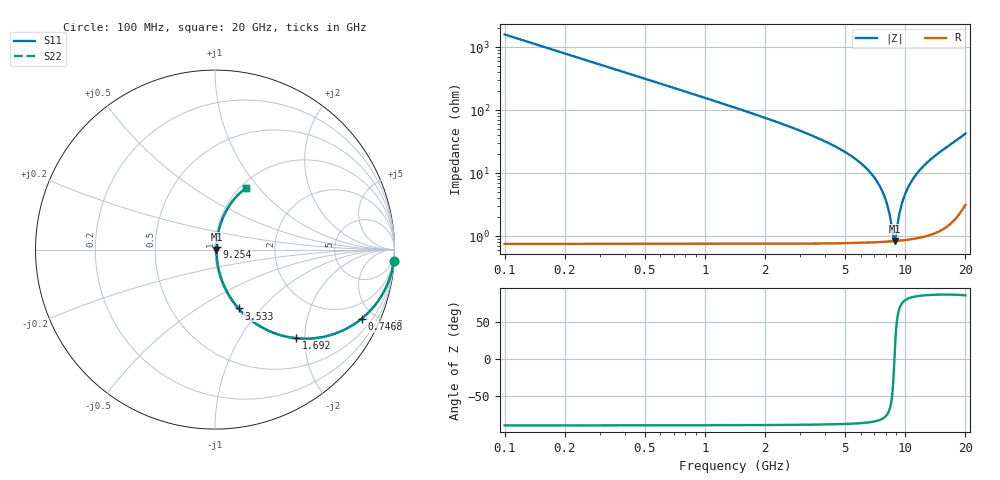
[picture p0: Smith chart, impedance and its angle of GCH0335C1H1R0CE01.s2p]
!Murata Part Number: GCH0335C1H1R0CE01
!These Parameters are Measured in Series Mode Connection
!Data Generated on Mar 13, 2026
!  o--ll--o
!Port1  Port2
!  o------o
!Operation Temp=25[degC], DC Bias Voltage=0[V]
!Freq. Start=100[MHz] Stop=20[GHz] 401[Steps]
# Hz S RI R 50
!Freq.(Hz) S11(Real) S11(Imag) S21(Real) S21(Imag) S12(Real) S12(Imag) S22(Real) S22(Imag)
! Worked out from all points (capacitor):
!   401 points, 100 MHz to 20 GHz, reference 50 ohm
!   read as one part in series: C = 1 pF near 199.5 MHz
!   lowest |Z| = 840 mohm at 8.856 GHz (marker M1)
!   series resonance near 8.845 GHz, so ESL is about 320 pH
!   S11 on the Smith chart (normalised r, x): 100 MHz: 1, -32; 746.8 MHz: 1.02, -4.23; 1.692 GHz: 1.02, -1.81; 3.533 GHz: 1.02, -0.76; 9.254 GHz: 1.02, +0.03; 20 GHz: 1.06, +0.85
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1e8  0.996 -0.0626  0.00396 0.0626  0.00396 0.0626  0.996 -0.0626
2.99e8  0.9656 -0.1816  0.0344 0.1816  0.0344 0.1816  0.9656 -0.1816
3.985e8  0.9404 -0.2358  0.0596 0.2358  0.0596 0.2358  0.9404 -0.2358
7.4675e8  0.8166 -0.3852  0.1834 0.3852  0.1834 0.3852  0.8166 -0.3852
1.1945e9  0.6306 -0.4797  0.3694 0.4797  0.3694 0.4797  0.6306 -0.4797
1.692e9  0.4518 -0.4935  0.5482 0.4935  0.5482 0.4935  0.4518 -0.4935
2.488e9  0.2611 -0.4328  0.7389 0.4328  0.7389 0.4328  0.2611 -0.4328
3.43325e9  0.1399 -0.3373  0.8601 0.3373  0.8601 0.3373  0.1399 -0.3373
3.53275e9  0.1312 -0.3277  0.8688 0.3277  0.8688 0.3277  0.1312 -0.3277
6.7665e9  0.0174 -0.0965  0.9826 0.0965  0.9826 0.0965  0.0174 -0.0965
7.9605e9  0.00959 -0.0381  0.9904 0.0381  0.9904 0.0381  0.00959 -0.0381
8.3585e9  0.00863 -0.0205  0.9914 0.0205  0.9914 0.0205  0.00863 -0.0205
8.7565e9  0.00831 -0.00366  0.9917 0.00366  0.9917 0.00366  0.00831 -0.00366
8.856e9  0.00832 0.000444  0.9917 -0.000444  0.9917 -0.000444  0.00832 0.000444
8.9555e9  0.00837 0.00451  0.9916 -0.00451  0.9916 -0.00451  0.00837 0.00451
9.254e9  0.0087 0.0165  0.9913 -0.0165  0.9913 -0.0165  0.0087 0.0165
9.60225e9  0.00943 0.03  0.9906 -0.03  0.9906 -0.03  0.00943 0.03
1.005e10  0.0109 0.0468  0.9891 -0.0468  0.9891 -0.0468  0.0109 0.0468
1.13435e10  0.0178 0.0923  0.9822 -0.0923  0.9822 -0.0923  0.0178 0.0923
1.338325e10  0.036 0.1571  0.964 -0.1571  0.964 -0.1571  0.036 0.1571
1.67165e10  0.0851 0.2529  0.9149 -0.2529  0.9149 -0.2529  0.0851 0.2529
2e10  0.1715 0.3418  0.8285 -0.3418  0.8285 -0.3418  0.1715 0.3418
